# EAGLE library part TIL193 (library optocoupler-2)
TEXAS INSTRUMENTS OPTO COUPLER
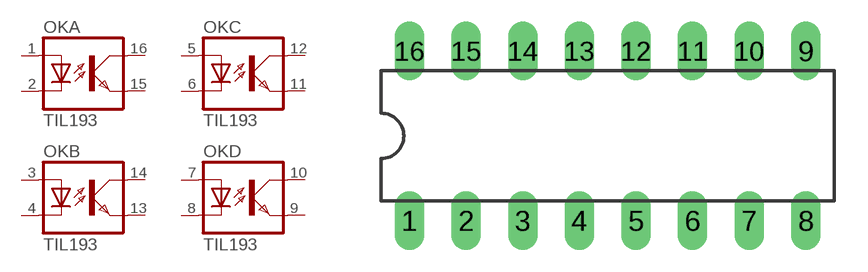
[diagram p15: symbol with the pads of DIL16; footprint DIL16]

Designator prefix OK; gates A=OK B=OK C=OK D=OK

## TIL193  [DIL16]
1  A:A  pas
2  A:C  pas
3  B:A  pas
4  B:C  pas
5  C:A  pas
6  C:C  pas
7  D:A  pas
8  D:C  pas
9  D:EMIT  pas
10  D:COL  pas
11  C:EMIT  pas
12  C:COL  pas
13  B:EMIT  pas
14  B:COL  pas
15  A:EMIT  pas
16  A:COL  pas

## Footprint DIL16 (pad centres in mm)
Dual In Line Package
drill 0.813 long: 1 -8.89,-3.81; 2 -6.35,-3.81; 3 -3.81,-3.81; 4 -1.27,-3.81; 5 1.27,-3.81; 6 3.81,-3.81; 7 6.35,-3.81; 8 8.89,-3.81; 9 8.89,3.81; 10 6.35,3.81; 11 3.81,3.81; 12 1.27,3.81; 13 -1.27,3.81; 14 -3.81,3.81; 15 -6.35,3.81; 16 -8.89,3.81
